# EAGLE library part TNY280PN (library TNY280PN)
Power Integrations TNY280PN Intelligent Power Switch, Off Line Switcher, 2550mA, 28.5W 8-Pin, DIPC Source: Datasheet
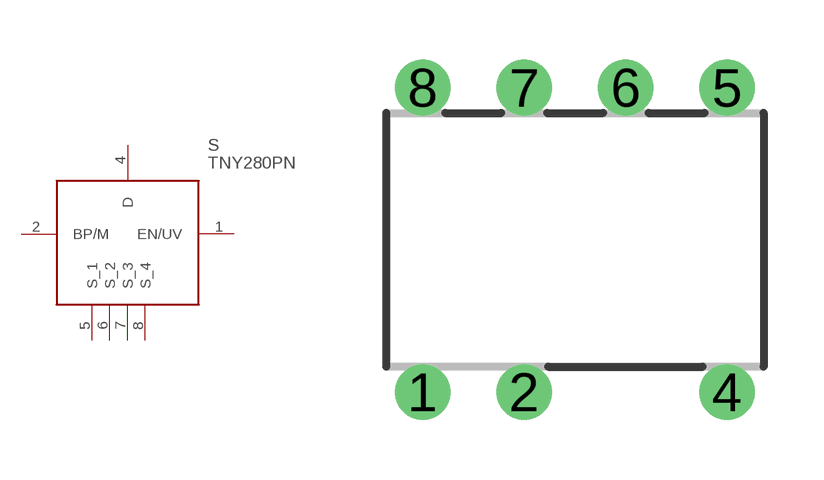
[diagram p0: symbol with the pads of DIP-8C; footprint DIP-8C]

Designator prefix S

## TNY280PN (Description: Power Integrations TNY280PN Intelligent Power Switch, Off Line Switcher, 2550mA, 28.5W 8-Pin, DIPC; Height: mm; Manufacturer_Name: Power Integrations; Manufacturer_Part_Number: TNY280PN; Mouser_Part_Number: 869-TNY280PN; Mouser_Price-Stock: https://www.mouser.co.uk/ProductDetail/Power-Integrations/TNY280PN?qs=WS5Jv%252B%252Bx1qW1eUCHvoKBfA%3D%3D)  [DIP-8C]
1  EN/UV
2  BP/M
4  D
5  S_1
6  S_2
7  S_3
8  S_4

## Footprint DIP-8C (pad centres in mm)
DIP-8C
drill 0.88 pad 1.38: 1 -1.27,-7.62; 2 1.27,-7.62; 4 6.35,-7.62; 5 6.35,0; 6 3.81,0; 7 1.27,0; 8 -1.27,0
